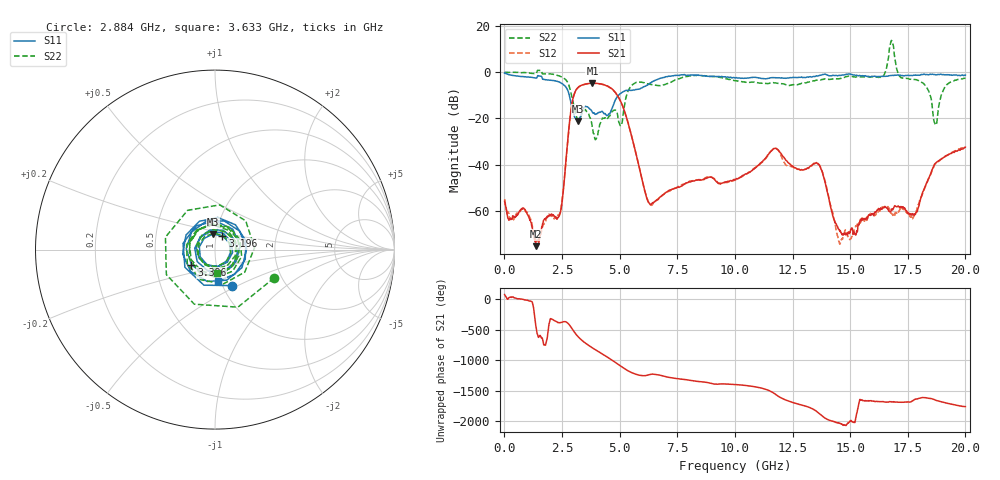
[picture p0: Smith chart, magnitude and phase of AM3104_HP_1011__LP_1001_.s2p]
!Created with skrf (http://scikit-rf.org).
# Hz S RI R 50.0
!freq ReS11 ImS11 ReS21 ImS21 ReS12 ImS12 ReS22 ImS22
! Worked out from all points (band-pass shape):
!   1601 points, 10 MHz to 20 GHz, reference 50 ohm
!   highest |S21| = -4.76 dB at 3.821 GHz (marker M1); lowest = -75.1 dB at 1.384 GHz (marker M2)
!   |S21| within 3 dB of the highest: 3.105 GHz to 4.724 GHz (1.619 GHz wide, 41.4 % of centre)
!   lowest |S11| = -21.2 dB at 3.183 GHz (marker M3), VSWR 1.19, Z = 48.1 + j8.36 ohm
!   |S11| at or under -10 dB: 2.818 GHz to 4.95 GHz (2.132 GHz wide, 54.9 % of centre)
!   |S22| runs from -29.2 to 13.7 dB; largest |S21 - S12| = 0.047
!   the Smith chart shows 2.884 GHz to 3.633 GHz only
!   S11 on the Smith chart (normalised r, x): 2.884 GHz: 1.10, -0.47; 3.196 GHz: 1.07, +0.17; 3.396 GHz: 0.76, -0.13; 3.633 GHz: 0.97, -0.35
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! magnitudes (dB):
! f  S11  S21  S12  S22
! 10 MHz  -0.4  -55.8  -54.8  0.0
! 1.384 GHz  -2.6  -75.1  -72.8  -0.6
! 2.409 GHz  -4.4  -61.2  -60.4  -1.8
! 2.884 GHz  -13.1  -16.8  -16.9  -8.8
! 3.183 GHz  -21.2  -6.8  -6.8  -20.6
! 3.196 GHz  -21.2  -6.6  -6.7  -20.7
! 3.346 GHz  -18.0  -5.7  -5.7  -18.4
! 3.396 GHz  -16.1  -5.5  -5.5  -17.0
! 3.633 GHz  -15.1  -5.0  -5.1  -17.6
! 3.821 GHz  -17.3  -4.8  -4.8  -24.2
! 4.958 GHz  -9.9  -10.9  -11.0  -21.3
! 6.207 GHz  -5.6  -55.3  -54.9  -5.0
! 6.682 GHz  -3.0  -54.6  -54.8  -5.8
! 10.01 GHz  -2.5  -46.5  -46.6  -3.7
! 11.72 GHz  -2.4  -33.0  -33.0  -4.6
! 13.34 GHz  -2.1  -40.2  -40.3  -4.0
! 13.77 GHz  -1.2  -42.5  -42.2  -3.2
! 14.57 GHz  -1.4  -68.8  -73.8  -2.7
! 16.68 GHz  -1.6  -60.0  -59.0  7.2
! 17.76 GHz  -1.3  -61.6  -62.2  -3.2
! 18.69 GHz  -1.1  -39.4  -39.7  -22.4
! 20 GHz  -1.3  -32.4  -32.3  -2.6
